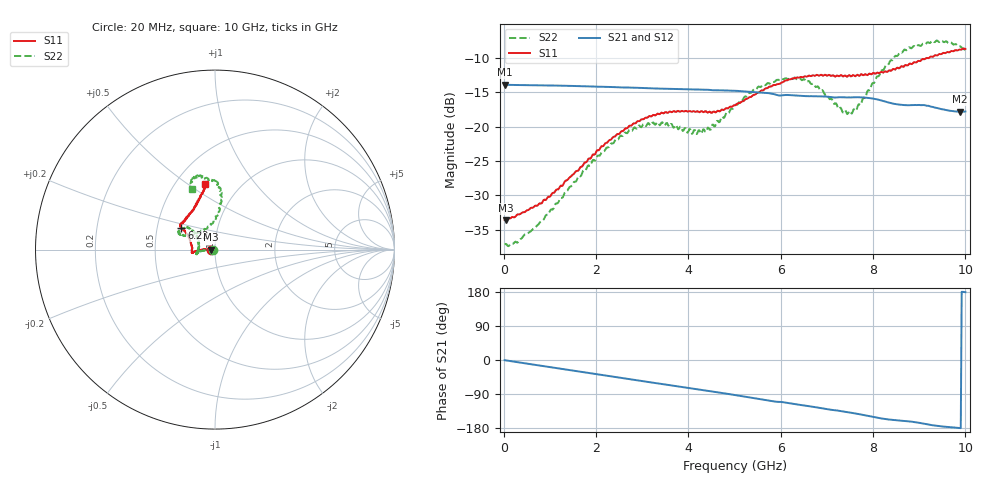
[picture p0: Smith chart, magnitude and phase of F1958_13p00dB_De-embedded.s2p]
! Integrated Device Technology
! Corporate Headquarters
! 6024 Silver Creek Valley Road
! San Jose, CA 95138  USA
! Phone:  1-408-284-8200
! Toll Free:  1-800-223-1366
! Webpage:  http://www.idt.com/
! Timing and RF Division
! 515 Groton Road, Suite 102
! Westford, MA 01886-6024
! Device:  F1958
! Description: 7-bit 0.25 dB Digital Step Attenuator
! Frequency:  0.001 -  6.000 GHz
! Package:  4x4 mm Thin QFN Plastic Package: 24 pin
! Ports:  2 RF, 12 DC
!  Pin  1  = D0
!  Pin  2  = VDD
!  Pin  3  = VMODE
!  Pin  4  = GND
!  Pin  5  = RF1  =  Port 1
!  Pin  6  = GND
!  Pin  7  = GND
!  Pin  8  = GND
!  Pin  9  = GND
!  Pin 10  = GND
!  Pin 11  = GND
!  Pin 12  = GND
!  Pin 13  = GND
!  Pin 14  = RF2  =  Port 2
!  Pin 15  = GND
!  Pin 16  = LE
!  Pin 17  = CLK
!  Pin 18  = DATA
!  Pin 19  = D6
!  Pin 20  = D5
!  Pin 21  = D4
!  Pin 22  = D3
!  Pin 23  = D2
!  Pin 24  = D1
! State:  52
! Atten State:  13.00 dB
! Voltage:  +3.30 Volts
! Current:  0.258 mA
! Data:  The device was measured on a F1958 evaluation board which has
!  individual transmission lines to the RF pins.  Data was collected
!  using a calibrated network analyzer.  The evaluation board was
!  de-embedded using Automatic Fixture Removal (AFR).
!  The reference plane is the edge of the package pin.
! Misc:
!  Action Tracker AT0419
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# GHz S dB R 50
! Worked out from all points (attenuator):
!   500 points, 20 MHz to 10 GHz, reference 50 ohm
!   highest |S21| = -13.87 dB at 20 MHz (marker M1); lowest = -17.8 dB at 9.88 GHz (marker M2)
!   lowest |S11| = -33.6 dB at 40 MHz (marker M3), VSWR 1.04, Z = 48 - j0.0833 ohm
!   |S11| at or under -10 dB: start of sweep to 9.155 GHz; 9.189477 GHz to 9.202163 GHz (12.69 MHz wide, 0.138 % of centre)
!   |S22| runs from -37.4 to -7.4 dB; largest |S21 - S12| = 0.0006
!   S11 on the Smith chart (normalised r, x): 20 MHz: 0.96, -0.00; 6.22 GHz: 0.67, +0.17; 10 GHz: 0.69, +0.58
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0.02  -33.58 -177.7  -13.87 -0.5  -13.87 -0.5  -37.17 -176.7
0.04  -33.60 -177.6  -13.88 -0.9  -13.88 -0.9  -37.06 -175.0
0.32  -32.77 178.2  -13.92 -6.1  -13.92 -6.1  -36.72 -179.5
0.72  -31.52 179.0  -13.96 -13.6  -13.96 -13.5  -34.41 -176.5
1.7  -25.78 179.8  -14.10 -31.6  -14.09 -31.6  -26.75 -176.6
2.6  -20.53 -176.7  -14.27 -48.2  -14.26 -48.2  -21.12 -172.9
2.92  -19.18 -174.1  -14.33 -54.1  -14.32 -54.1  -19.84 -169.8
3.36  -18.16 -171.9  -14.44 -62.2  -14.44 -62.3  -19.61 -165.6
4.3  -17.77 -178.1  -14.59 -79.3  -14.60 -79.3  -20.72 165.8
4.54  -17.79 175.8  -14.69 -83.7  -14.70 -83.8  -19.71 157.4
5.02  -16.86 161.9  -14.76 -92.7  -14.77 -92.7  -16.76 141.0
5.54  -14.96 151.3  -15.00 -102.6  -15.01 -102.6  -14.18 142.0
6.22  -13.08 147.3  -15.41 -114.9  -15.42 -114.8  -12.90 153.2
6.68  -12.54 145.0  -15.55 -123.1  -15.57 -123.0  -13.76 155.6
7.32  -12.52 139.4  -15.71 -135.2  -15.72 -135.1  -17.53 135.0
7.5  -12.54 136.3  -15.73 -138.6  -15.74 -138.5  -17.71 116.9
7.68  -12.51 133.4  -15.70 -142.4  -15.70 -142.4  -16.78 99.3
8.34  -11.81 117.6  -16.48 -157.0  -16.48 -157.1  -10.85 82.7
8.68  -11.15 110.8  -16.83 -160.9  -16.85 -160.9  -8.75 87.2
9.26  -9.77 103.0  -17.08 -171.7  -17.08 -171.7  -7.61 100.2
9.88  -8.74 99.0  -17.81 -179.6  -17.83 -179.5  -8.28 109.9
10  -8.65 98.8  -17.77 178.9  -17.81 179.0  -8.82 110.8
